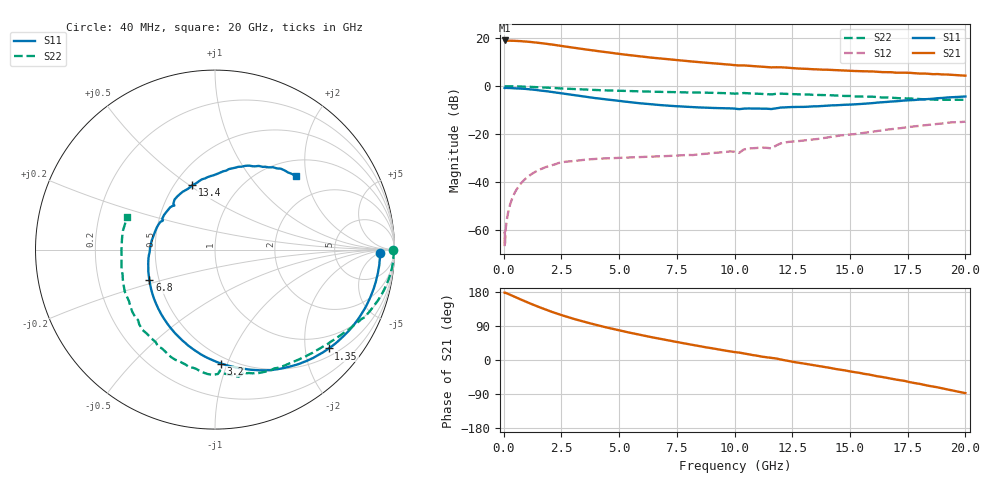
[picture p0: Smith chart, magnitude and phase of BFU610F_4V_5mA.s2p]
! Filename:  P:\Prog\Test\Noise\ATS_data\Testdata_Net\SplitFiles\BFU610_2W_A5_HighFreq_4V_5mA_D.s2p
! Date/Time: Wed 10/Aug/2011 16:57:51
! BFU610_2W_A5_HighFreq_4V_1mA_10mA_Bias3_R.s2p
! MDIF S-parameter v. bias file
! BFU610_2W_A5_HighFreq_4V_1mA_10mA
! Date/time Mon Aug 08 14:12:42 2011
! VAR V_out= 4.0000
! VAR I_out= 4.9900
! VAR V_in= 0.8854
! VAR I_in= 0.0392
! Device data file deembeded for feedlines and parallel
! Original file: \SplitFiles\BFU610_2W_A5_HighFreq_4V_5mA_R.s2p
! Feed-files: PR003V01_101208_Feed1.s2p, PR003V01_101208_Feed2.s2p
! Parallel-file: PR003V01_101208_Par.s2p
# MHz S MA R 50
!  Freq-MHz  S11-mag  S11-arg  S21-mag  S21-arg  S12-mag  S12-arg  S22-mag  S22-arg
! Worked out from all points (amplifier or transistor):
!   167 points, 40 MHz to 20 GHz, reference 50 ohm
!   highest |S21| = 19.1 dB at 40 MHz (marker M1)
!   |S21| within 3 dB of that: start of sweep to 3.008 GHz
!   unconditionally stable (mu >= 1): 5.477 GHz to 16.43 GHz
!   at 550 MHz: K = 0.04, MSG = 31.0 dB, |S12| = -43.2 dB
!   at 4.2 GHz: K = 0.74, MSG = 22.3 dB, |S12| = -30.2 dB
!   at 20 GHz: K = 0.74, MSG = 9.6 dB, |S12| = -14.8 dB
!   S11 on the Smith chart (normalised r, x): 40 MHz: 23, -5; 1.35 GHz: 0.67, -2.52; 3.2 GHz: 0.45, -0.95; 6.8 GHz: 0.44, -0.18; 13.4 GHz: 0.61, +0.51; 20 GHz: 1.35, +1.75
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40  0.9195 -1.1  8.968 177.8  0.0004642 85.3  0.993 -0.2
50  0.9123 -1.4  8.923 178.0  0.0009227 53.9  0.994 -0.4
60  0.9223 -1.6  8.938 177.3  0.0005342 77.2  0.9946 -0.5
140  0.9193 -4.3  8.885 175.8  0.001693 89.4  0.9952 -1.6
380  0.9128 -11.9  8.835 169.4  0.004761 86.2  0.9932 -4.5
900  0.8812 -27.9  8.558 155.5  0.01127 75.8  0.9786 -10.6
1350  0.8397 -41.0  8.169 144.1  0.01624 67.7  0.9589 -15.6
1750  0.7967 -52.0  7.75 134.6  0.01997 61.3  0.9385 -19.6
2200  0.7457 -63.7  7.245 124.6  0.0233 55.5  0.9156 -24.0
2700  0.6857 -75.9  6.685 114.8  0.02674 48.3  0.8836 -28.0
3200  0.6357 -87.0  6.151 105.7  0.02819 44.0  0.8609 -31.9
3400  0.6161 -91.3  5.967 102.4  0.0289 42.6  0.8527 -33.3
4100  0.5546 -105.7  5.37 91.2  0.03086 38.2  0.8266 -38.1
4900  0.4967 -121.0  4.779 79.6  0.03214 35.3  0.8031 -43.4
5800  0.4456 -137.5  4.243 67.7  0.03331 33.7  0.7815 -49.3
6800  0.4033 -155.0  3.759 55.6  0.03457 33.6  0.7617 -55.7
8600  0.3586 175.4  3.136 35.4  0.03852 37.6  0.7355 -67.5
10200  0.3322 150.8  2.699 19.6  0.04072 42.4  0.7041 -76.8
12000  0.3584 128.9  2.473 1.3  0.06439 47.2  0.6986 -91.1
13400  0.3799 109.6  2.253 -13.4  0.07762 37.4  0.6606 -104.5
16800  0.4795 74.2  1.954 -49.4  0.1274 18.9  0.5758 -143.3
20000  0.6093 42.1  1.654 -87.5  0.182 -12.6  0.5205 159.8
